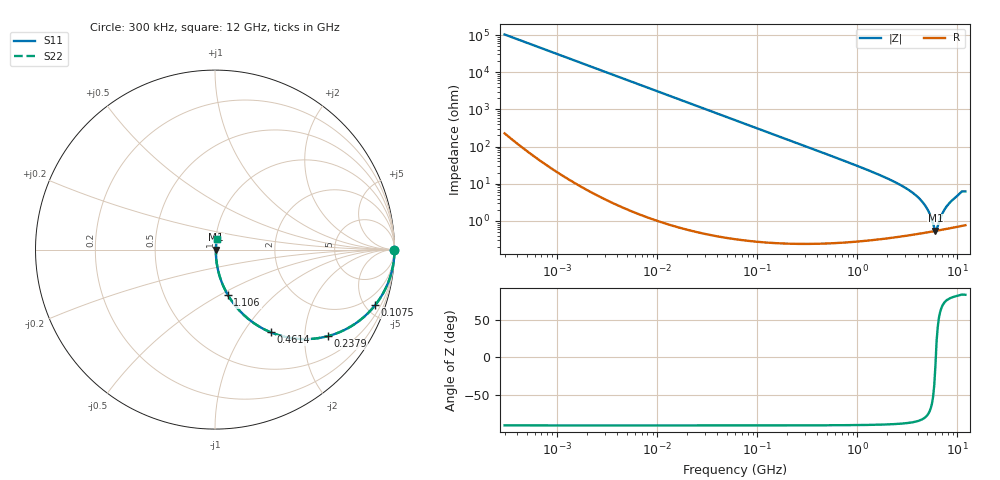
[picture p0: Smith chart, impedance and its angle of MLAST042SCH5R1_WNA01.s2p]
! MLAST042SCH5R1_WNA01  S-PARAMETER MODEL  ( General Type )
! Model Generated by TAIYO YUDEN Corporation (http://www.ty-top.com)
! Version 1.0
! TAIYO YUDEN Control No. 150820
! Copyright(c) 2015 TAIYO YUDEN CO.,LTD. All Rights Reserved.
! Product Description (link to TY-COMPAS)
! https://ds.yuden.co.jp/TYCOMPAS/or/detail?pn=MLAST042SCH5R1BWNA01&u=M
! Products Name : Multilayer Ceramic Capacitors
! Characteristics :
!  Capacitance : 5.1 pF , Rated Voltage : 25V , TCC : CH / C0H
!  Case Size : 0.4 x 0.2 / 0.016 x 0.008 [mm/inch] , Thickness : 0.2 / 0.008 [mm/inch]
!  (Conditions: Temperature = 25 degC , DC Bias Current/Voltage = 0A / 0V)
! External Node Assignments :
!  1  o---| |---o  2
! GND o---------o GND
! Frequency Range : 0.3MHz  -  12000MHz  [ 401 STEP ]
# MHz S RI R 50
! Freq[MHz].  S11 Real  S11 Imag  S21 Real  S21 Imag  S12 Real  S12 Imag  S22 Real  S22 Imag
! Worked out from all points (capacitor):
!   401 points, 300 kHz to 12 GHz, reference 50 ohm
!   read as one part in series: C = 5.12 pF near 316.3 kHz
!   lowest |Z| = 547 mohm at 6.026 GHz (marker M1)
!   series resonance near 6.077 GHz, so ESL is about 130 pH
!   S11 on the Smith chart (normalised r, x): 300 kHz: open; 107.5 MHz: 1.01, -5.78; 237.9 MHz: 1.00, -2.61; 461.4 MHz: 1.00, -1.34; 1.106 GHz: 1.01, -0.54; 12 GHz: 1.02, +0.12
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0.3  1 -0.000965  3.04e-06 0.000965  3.04e-06 0.000965  1 -0.000965
1.769972  1 -0.00569  3.5e-05 0.00569  3.5e-05 0.00569  1 -0.00569
10.44266  0.9989 -0.0336  0.00114 0.0336  0.00114 0.0336  0.9989 -0.0336
27.82928  0.992 -0.0888  0.00799 0.0888  0.00799 0.0888  0.992 -0.0888
60  0.964 -0.186  0.036 0.186  0.036 0.186  0.964 -0.186
107.4644  0.893 -0.3087  0.107 0.3087  0.107 0.3087  0.893 -0.3087
237.9135  0.6297 -0.4819  0.3703 0.4819  0.3703 0.4819  0.6297 -0.4819
353.9943  0.434 -0.4942  0.566 0.4942  0.566 0.4942  0.434 -0.4942
461.3684  0.3105 -0.4609  0.6895 0.4609  0.6895 0.4609  0.3105 -0.4609
704.9044  0.1607 -0.3643  0.8393 0.3643  0.8393 0.3643  0.1607 -0.3643
1105.905  0.0711 -0.2518  0.9289 0.2518  0.9289 0.2518  0.0711 -0.2518
2088.533  0.0202 -0.1283  0.9798 0.1283  0.9798 0.1283  0.0202 -0.1283
3190.978  0.00896 -0.0698  0.991 0.0698  0.991 0.0698  0.00896 -0.0698
4270.516  0.00592 -0.0367  0.9941 0.0367  0.9941 0.0367  0.00592 -0.0367
5006.236  0.00531 -0.02  0.9947 0.02  0.9947 0.02  0.00531 -0.02
5715.274  0.00527 -0.00651  0.9947 0.00651  0.9947 0.00651  0.00527 -0.00651
6026.253  0.00536 -0.000968  0.9946 0.000968  0.9946 0.000968  0.00536 -0.000968
6354.153  0.00552 0.00464  0.9945 -0.00464  0.9945 -0.00464  0.00552 0.00464
7064.448  0.006 0.0146  0.994 -0.0146  0.994 -0.0146  0.006 0.0146
8064.993  0.00689 0.0264  0.9931 -0.0264  0.9931 -0.0264  0.00689 0.0264
10511.28  0.00996 0.0531  0.99 -0.0531  0.99 -0.0531  0.00996 0.0531
12000  0.0114 0.0608  0.9886 -0.0608  0.9886 -0.0608  0.0114 0.0608
